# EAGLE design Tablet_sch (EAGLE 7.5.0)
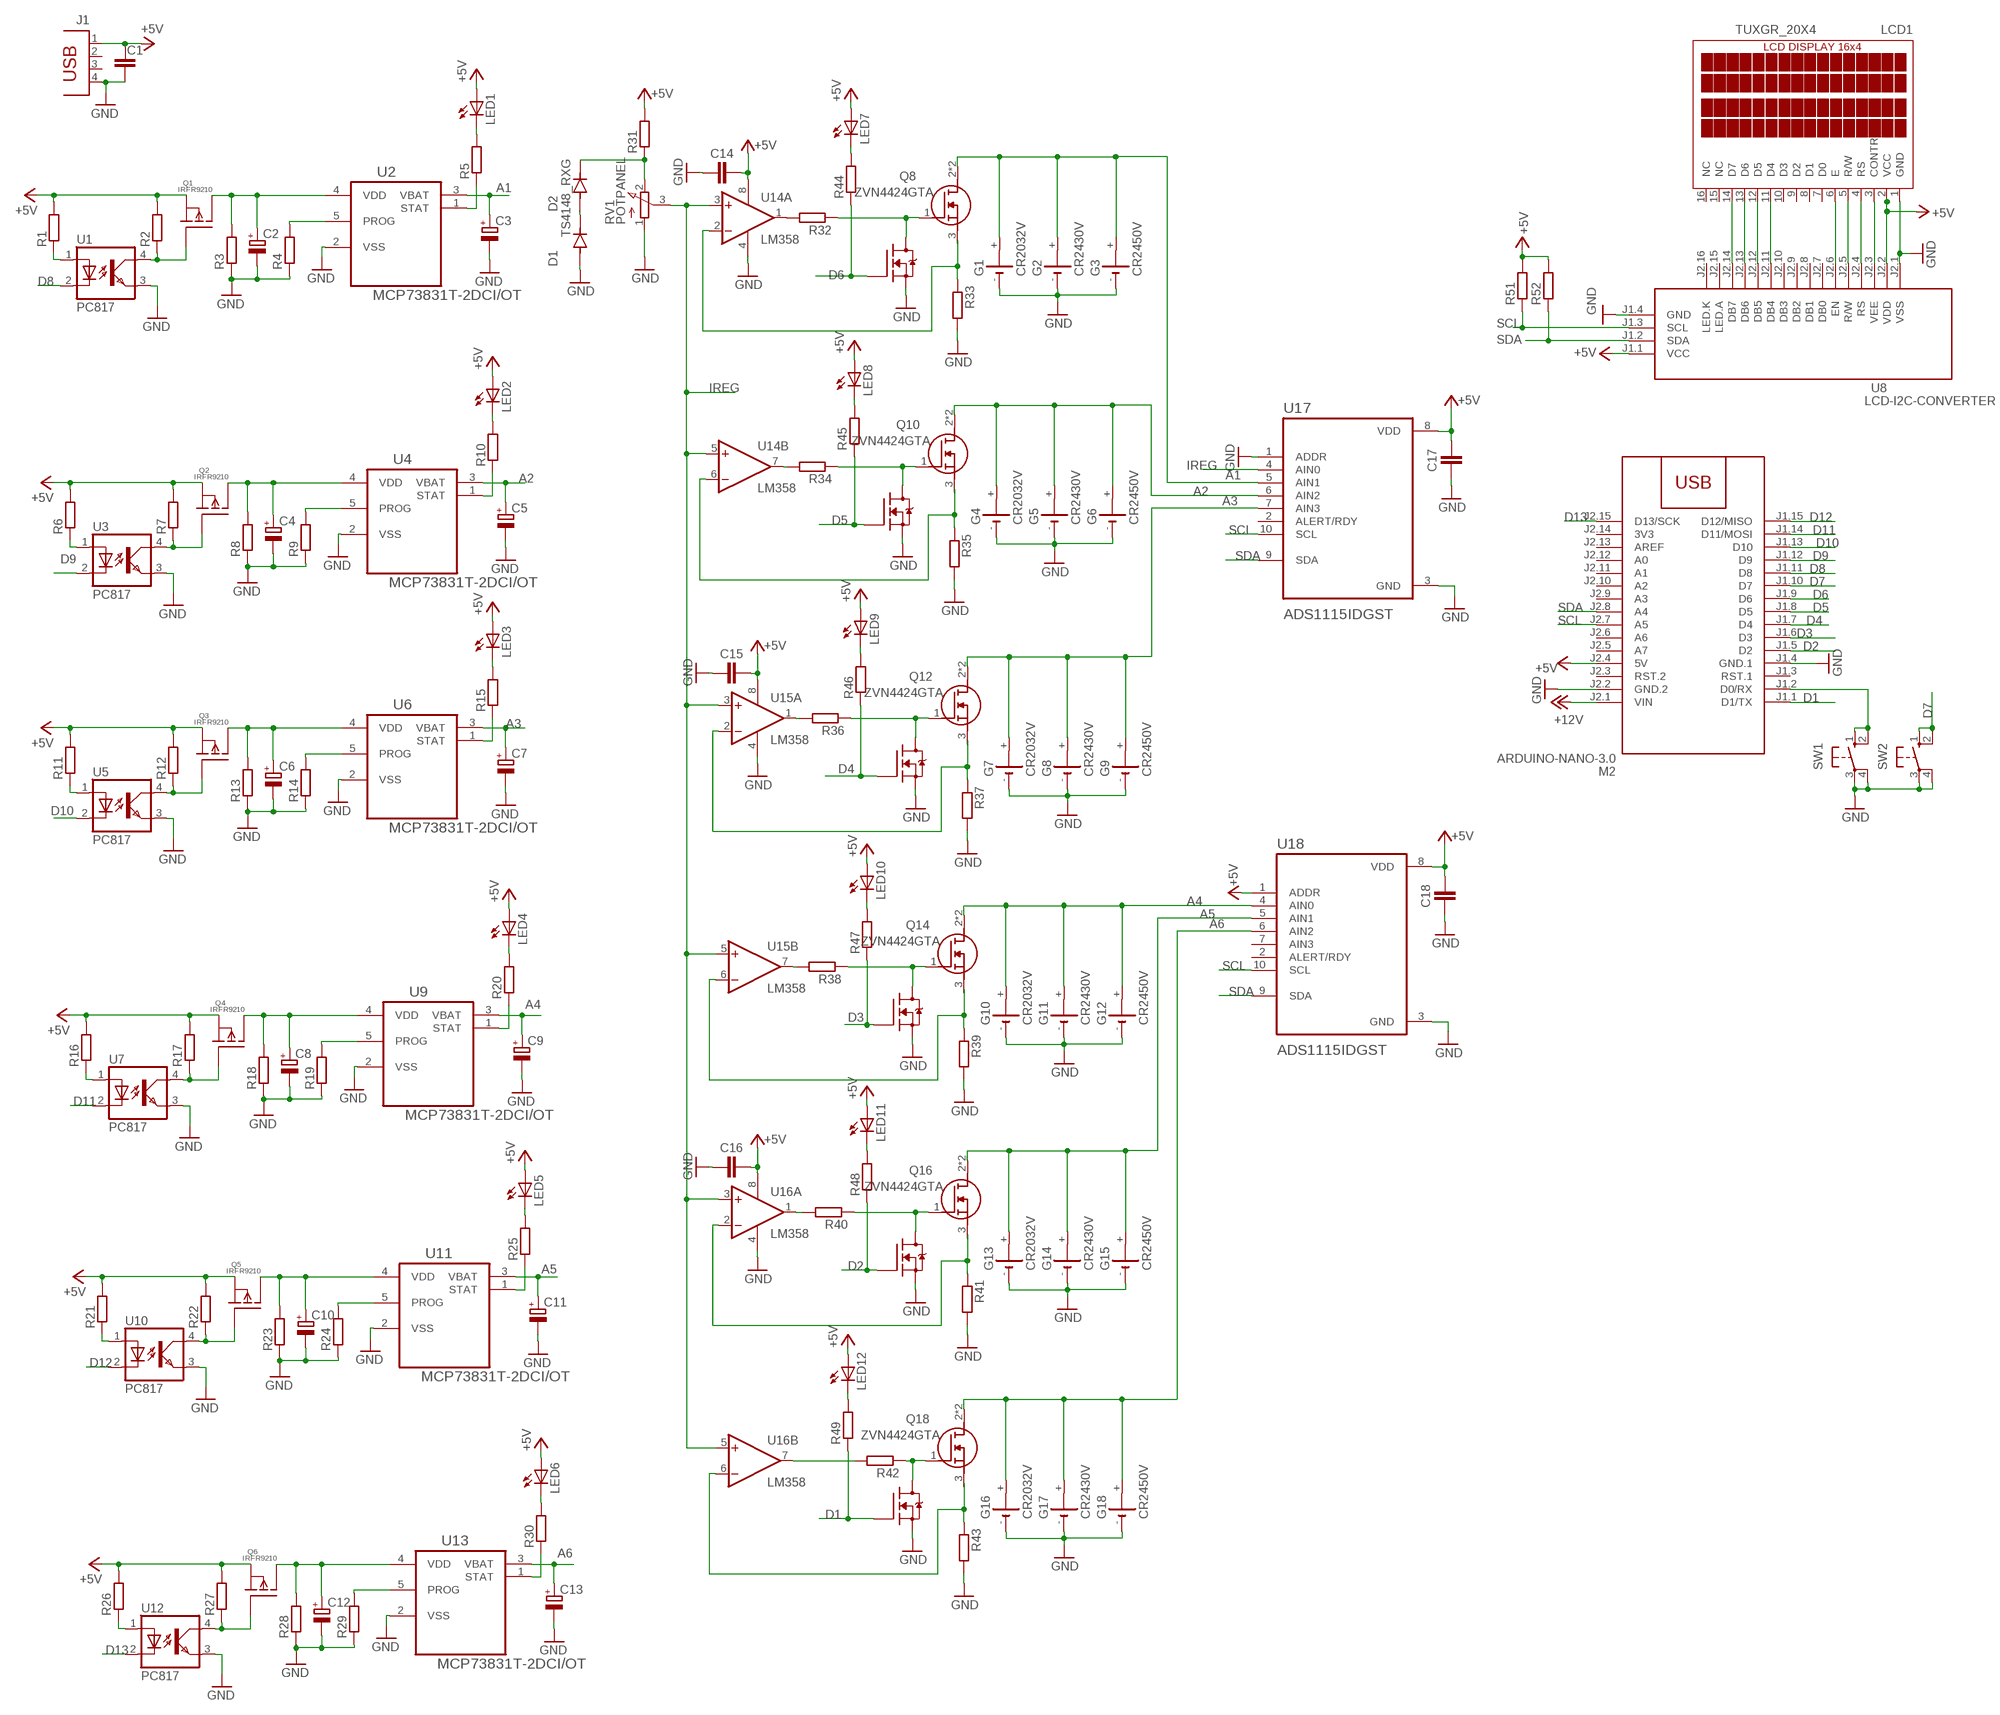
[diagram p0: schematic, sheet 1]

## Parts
C1  C-EUC1206  [C1206]
C2  CPOL-EUSMCB  [SMC_B]
C3  CPOL-EUSMCB  [SMC_B]
C4  CPOL-EUSMCB  [SMC_B]
C5  CPOL-EUSMCB  [SMC_B]
C6  CPOL-EUSMCB  [SMC_B]
C7  CPOL-EUSMCB  [SMC_B]
C8  CPOL-EUSMCB  [SMC_B]
C9  CPOL-EUSMCB  [SMC_B]
C10  CPOL-EUSMCB  [SMC_B]
C11  CPOL-EUSMCB  [SMC_B]
C12  CPOL-EUSMCB  [SMC_B]
C13  CPOL-EUSMCB  [SMC_B]
C14  C-EUC1206  [C1206]
C15  C-EUC1206  [C1206]
C16  C-EUC1206  [C1206]
C17  C-EUC1206  [C1206]
C18  C-EUC1206  [C1206]
D1  TS4148_RXG  [DIO_TS4148_RXG]
D2  TS4148_RXG  [DIO_TS4148_RXG]
G1  CR2032V  [CR2032V]
G2  CR2430V  [CR2430V]
G3  CR2450V  [CR2450V]
G4  CR2032V  [CR2032V]
G5  CR2430V  [CR2430V]
G6  CR2450V  [CR2450V]
G7  CR2032V  [CR2032V]
G8  CR2430V  [CR2430V]
G9  CR2450V  [CR2450V]
G10  CR2032V  [CR2032V]
G11  CR2430V  [CR2430V]
G12  CR2450V  [CR2450V]
G13  CR2032V  [CR2032V]
G14  CR2430V  [CR2430V]
G15  CR2450V  [CR2450V]
G16  CR2032V  [CR2032V]
G17  CR2430V  [CR2430V]
G18  CR2450V  [CR2450V]
J1  PN87520  [PN87520]
LCD1  TUXGR_20X4  [TUXGR_20X4]
LED1  LED5MM  [LED5MM]
LED2  LED5MM  [LED5MM]
LED3  LED5MM  [LED5MM]
LED4  LED5MM  [LED5MM]
LED5  LED5MM  [LED5MM]
LED6  LED5MM  [LED5MM]
LED7  LED5MM  [LED5MM]
LED8  LED5MM  [LED5MM]
LED9  LED5MM  [LED5MM]
LED10  LED5MM  [LED5MM]
LED11  LED5MM  [LED5MM]
LED12  LED5MM  [LED5MM]
M2  ARDUINO-NANO-3.0  [ARDUINO-NANO-3.0]
Q1  IRFR9210  [D2PACK]
Q2  IRFR9210  [D2PACK]
Q3  IRFR9210  [D2PACK]
Q4  IRFR9210  [D2PACK]
Q5  IRFR9210  [D2PACK]
Q6  IRFR9210  [D2PACK]
Q7  ZVN3310F  [SOT23]
Q8  ZVN4424GTA  [ZVN4424GTA]
Q9  ZVN3310F  [SOT23]
Q10  ZVN4424GTA  [ZVN4424GTA]
Q11  ZVN3310F  [SOT23]
Q12  ZVN4424GTA  [ZVN4424GTA]
Q13  ZVN3310F  [SOT23]
Q14  ZVN4424GTA  [ZVN4424GTA]
Q15  ZVN3310F  [SOT23]
Q16  ZVN4424GTA  [ZVN4424GTA]
Q17  ZVN3310F  [SOT23]
Q18  ZVN4424GTA  [ZVN4424GTA]
R1  R-EU_R1206  [R1206]
R2  R-EU_R1206  [R1206]
R3  R-EU_R1206  [R1206]
R4  R-EU_R1206  [R1206]
R5  R-EU_R1206  [R1206]
R6  R-EU_R1206  [R1206]
R7  R-EU_R1206  [R1206]
R8  R-EU_R1206  [R1206]
R9  R-EU_R1206  [R1206]
R10  R-EU_R1206  [R1206]
R11  R-EU_R1206  [R1206]
R12  R-EU_R1206  [R1206]
R13  R-EU_R1206  [R1206]
R14  R-EU_R1206  [R1206]
R15  R-EU_R1206  [R1206]
R16  R-EU_R1206  [R1206]
R17  R-EU_R1206  [R1206]
R18  R-EU_R1206  [R1206]
R19  R-EU_R1206  [R1206]
R20  R-EU_R1206  [R1206]
R21  R-EU_R1206  [R1206]
R22  R-EU_R1206  [R1206]
R23  R-EU_R1206  [R1206]
R24  R-EU_R1206  [R1206]
R25  R-EU_R1206  [R1206]
R26  R-EU_R1206  [R1206]
R27  R-EU_R1206  [R1206]
R28  R-EU_R1206  [R1206]
R29  R-EU_R1206  [R1206]
R30  R-EU_R1206  [R1206]
R31  R-EU_R1206  [R1206]
R32  R-EU_R1206  [R1206]
R33  R-EU_R2512  [R2512]
R34  R-EU_R1206  [R1206]
R35  R-EU_R2512  [R2512]
R36  R-EU_R1206  [R1206]
R37  R-EU_R2512  [R2512]
R38  R-EU_R1206  [R1206]
R39  R-EU_R2512  [R2512]
R40  R-EU_R1206  [R1206]
R41  R-EU_R2512  [R2512]
R42  R-EU_R1206  [R1206]
R43  R-EU_R2512  [R2512]
R44  R-EU_R1206  [R1206]
R45  R-EU_R1206  [R1206]
R46  R-EU_R1206  [R1206]
R47  R-EU_R1206  [R1206]
R48  R-EU_R1206  [R1206]
R49  R-EU_R1206  [R1206]
R51  R-EU_R1206  [R1206]
R52  R-EU_R1206  [R1206]
RV1  POTPANEL  [POTPANELP231]
SW1  40-XX  [B3F-40XX]
SW2  40-XX  [B3F-40XX]
U1  PC817  [DIL04]
U2  MCP73831T-2DCI/OT  [SOT95P270X145-5N]
U3  PC817  [DIL04]
U4  MCP73831T-2DCI/OT  [SOT95P270X145-5N]
U5  PC817  [DIL04]
U6  MCP73831T-2DCI/OT  [SOT95P270X145-5N]
U7  PC817  [DIL04]
U8  LCD-I2C-CONVERTER  [LCD-I2C-CONVERTER]
U9  MCP73831T-2DCI/OT  [SOT95P270X145-5N]
U10  PC817  [DIL04]
U11  MCP73831T-2DCI/OT  [SOT95P270X145-5N]
U12  PC817  [DIL04]
U13  MCP73831T-2DCI/OT  [SOT95P270X145-5N]
U14  LM358  OPA2134PA  [DIL08]
U15  LM358  OPA2134PA  [DIL08]
U16  LM358  OPA2134PA  [DIL08]
U17  ADS1115IDGST  [SOP50P490X110-10N]
U18  ADS1115IDGST  [SOP50P490X110-10N]

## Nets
+5V: C1.1 C14.1 C15.1 C16.1 C17.1 C18.1 J1.1 LCD1.2(VCC) LED1.A LED2.A LED3.A LED4.A LED5.A LED6.A LED7.A LED8.A LED9.A LED10.A LED11.A LED12.A M2.J2.4(5V) Q1.3(S) Q2.3(S) Q3.3(S) Q4.3(S) Q5.3(S) Q6.3(S) R1.2 R2.2 R6.2 R7.2 R11.2 R12.2 R16.2 R17.2 R21.2 R22.2 R26.2 R27.2 R31.2 R51.2 R52.2 U8.J1.1(VCC) U8.J2.2(VDD) U14.8(A:V+) U15.8(A:V+) U16.8(A:V+) U17.8(VDD) U18.1(ADDR) U18.8(VDD)
+12V: M2.J2.1(VIN)
A1: C3.+ G1.+ G2.+ G3.+ Q8.2(D) Q8.4(D) U2.3(VBAT) U17.5(AIN1)
A2: C5.+ G4.+ G5.+ G6.+ Q10.2(D) Q10.4(D) U4.3(VBAT) U17.6(AIN2)
A3: C7.+ G7.+ G8.+ G9.+ Q12.2(D) Q12.4(D) U6.3(VBAT) U17.7(AIN3)
A4: C9.+ G10.+ G11.+ G12.+ Q14.2(D) Q14.4(D) U9.3(VBAT) U18.4(AIN0)
A5: C11.+ G13.+ G14.+ G15.+ Q16.2(D) Q16.4(D) U11.3(VBAT) U18.5(AIN1)
A6: C13.+ G16.+ G17.+ G18.+ Q18.2(D) Q18.4(D) U13.3(VBAT) U18.6(AIN2)
D1: M2.J1.1(D1/TX) Q17.2(G) R49.1
D2: M2.J1.5(D2) Q15.2(G) R48.1
D3: M2.J1.6(D3) Q13.2(G) R47.1
D4: M2.J1.7(D4) Q11.2(G) R46.1
D5: M2.J1.8(D5) Q9.2(G) R45.1
D6: M2.J1.9(D6) Q7.2(G) R44.1
D7: M2.J1.10(D7) SW2.1(S) SW2.2(S1)
D8: M2.J1.11(D8) U1.2(C)
D9: M2.J1.12(D9) U3.2(C)
D10: M2.J1.13(D10) U5.2(C)
D11: M2.J1.14(D11/MOSI) U7.2(C)
D12: M2.J1.15(D12/MISO) U10.2(C)
D13: M2.J2.15(D13/SCK) U12.2(C)
GND: C1.2 C2.- C3.- C4.- C5.- C6.- C7.- C8.- C9.- C10.- C11.- C12.- C13.- C14.2 C15.2 C16.2 C17.2 C18.2 D1.A G1.- G2.- G3.- G4.- G5.- G6.- G7.- G8.- G9.- G10.- G11.- G12.- G13.- G14.- G15.- G16.- G17.- G18.- J1.4 LCD1.1(GND) M2.J1.4(GND.1) M2.J2.2(GND.2) Q7.3(S) Q9.3(S) Q11.3(S) Q13.3(S) Q15.3(S) Q17.3(S) R3.1 R4.1 R8.1 R9.1 R13.1 R14.1 R18.1 R19.1 R23.1 R24.1 R28.1 R29.1 R33.2 R35.2 R37.2 R39.2 R41.2 R43.2 RV1.1(A) SW1.3(P) SW1.4(P1) SW2.3(P) SW2.4(P1) U1.3(EMIT) U2.2(VSS) U3.3(EMIT) U4.2(VSS) U5.3(EMIT) U6.2(VSS) U7.3(EMIT) U8.J1.4(GND) U8.J2.1(VSS) U9.2(VSS) U10.3(EMIT) U11.2(VSS) U12.3(EMIT) U13.2(VSS) U14.4(A:V-) U15.4(A:V-) U16.4(A:V-) U17.1(ADDR) U17.3(GND) U18.3(GND)
IREG: RV1.3(S) U14.3(A:+IN) U14.5(B:+IN) U15.3(A:+IN) U15.5(B:+IN) U16.3(A:+IN) U16.5(B:+IN) U17.4(AIN0)
N$1: LCD1.14(D7) U8.J2.14(DB7)
N$2: LCD1.13(D6) U8.J2.13(DB6)
N$3: LCD1.12(D5) U8.J2.12(DB5)
N$4: LCD1.11(D4) U8.J2.11(DB4)
N$5: LCD1.6(E) U8.J2.6(EN)
N$6: LCD1.5(R/W) U8.J2.5(R/W)
N$7: LCD1.4(RS) U8.J2.4(RS)
N$8: M2.J1.2(D0/RX) SW1.1(S) SW1.2(S1)
N$9: R1.1 U1.1(A)
N$10: LCD1.3(CONTR) U8.J2.3(VEE)
N$11: LED6.K(C) R30.2
N$12: Q1.1(G) R2.1 U1.4(COL)
N$13: C2.+ Q1.2(D) R3.2 U2.4(VDD)
N$14: R5.1 U2.1(STAT)
N$15: R4.2 U2.5(PROG)
N$16: LED1.K(C) R5.2
N$18: R6.1 U3.1(A)
N$20: Q2.1(G) R7.1 U3.4(COL)
N$21: C4.+ Q2.2(D) R8.2 U4.4(VDD)
N$22: R9.2 U4.5(PROG)
N$24: R10.1 U4.1(STAT)
N$25: LED2.K(C) R10.2
N$26: R11.1 U5.1(A)
N$28: Q3.1(G) R12.1 U5.4(COL)
N$29: C6.+ Q3.2(D) R13.2 U6.4(VDD)
N$30: R14.2 U6.5(PROG)
N$32: R15.1 U6.1(STAT)
N$33: LED3.K(C) R15.2
N$34: R16.1 U7.1(A)
N$36: Q4.1(G) R17.1 U7.4(COL)
N$37: C8.+ Q4.2(D) R18.2 U9.4(VDD)
N$38: R19.2 U9.5(PROG)
N$40: R20.1 U9.1(STAT)
N$41: LED4.K(C) R20.2
N$42: R21.1 U10.1(A)
N$44: Q5.1(G) R22.1 U10.4(COL)
N$45: C10.+ Q5.2(D) R23.2 U11.4(VDD)
N$46: R24.2 U11.5(PROG)
N$48: R25.1 U11.1(STAT)
N$49: LED5.K(C) R25.2
N$50: R26.1 U12.1(A)
N$52: Q6.1(G) R27.1 U12.4(COL)
N$53: C12.+ Q6.2(D) R28.2 U13.4(VDD)
N$54: R29.2 U13.5(PROG)
N$56: R30.1 U13.1(STAT)
N$58: D2.C(K) R31.1 RV1.2(E)
N$59: D1.C(K) D2.A
N$60: R32.2 U14.1(A:OUT)
N$61: Q7.1(D) Q8.1(G) R32.1
N$62: Q8.3(S) R33.1 U14.2(A:-IN)
N$64: R34.2 U14.7(B:OUT)
N$65: Q9.1(D) Q10.1(G) R34.1
N$66: Q10.3(S) R35.1 U14.6(B:-IN)
N$68: R36.2 U15.1(A:OUT)
N$69: Q11.1(D) Q12.1(G) R36.1
N$70: Q12.3(S) R37.1 U15.2(A:-IN)
N$72: R38.2 U15.7(B:OUT)
N$73: Q13.1(D) Q14.1(G) R38.1
N$74: Q14.3(S) R39.1 U15.6(B:-IN)
N$76: R40.2 U16.1(A:OUT)
N$77: Q15.1(D) Q16.1(G) R40.1
N$78: Q16.3(S) R41.1 U16.2(A:-IN)
N$80: R42.2 U16.7(B:OUT)
N$81: Q17.1(D) Q18.1(G) R42.1
N$82: Q18.3(S) R43.1 U16.6(B:-IN)
N$84: LED8.K(C) R45.2
N$85: LED10.K(C) R47.2
N$86: LED11.K(C) R48.2
N$87: LED12.K(C) R49.2
N$90: LED9.K(C) R46.2
N$91: LED7.K(C) R44.2
SCL: M2.J2.7(A5) R51.1 U8.J1.3(SCL) U17.10(SCL) U18.10(SCL)
SDA: M2.J2.8(A4) R52.1 U8.J1.2(SDA) U17.9(SDA) U18.9(SDA)
Unconnected: G1.+@1(+) G2.+@1(+) G3.+@1(+) G4.+@1(+) G5.+@1(+) G6.+@1(+) G7.+@1(+) G8.+@1(+) G9.+@1(+) G10.+@1(+) G11.+@1(+) G12.+@1(+) G13.+@1(+) G14.+@1(+) G15.+@1(+) G16.+@1(+) G17.+@1(+) G18.+@1(+) J1.2 J1.3 LCD1.7(D0) LCD1.8(D1) LCD1.9(D2) LCD1.10(D3) LCD1.15(NC) LCD1.16(NC) M2.J1.3(RST.1) M2.J2.3(RST.2) M2.J2.5(A7) M2.J2.6(A6) M2.J2.9(A3) M2.J2.10(A2) M2.J2.11(A1) M2.J2.12(A0) M2.J2.13(AREF) U8.J2.7(DB0) U8.J2.8(DB1) U8.J2.9(DB2) U8.J2.10(DB3) U8.J2.15(LED.A) U8.J2.16(LED.K) U17.2(ALERT/RDY) U18.2(ALERT/RDY) U18.7(AIN3)

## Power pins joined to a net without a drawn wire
3V3: M2.J2.14(3V3)

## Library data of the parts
C1 C14-C18 = rcl:C-EU: CAPACITOR, European symbol
C2-C13 = rcl:CPOL-EU: POLARIZED CAPACITOR, European symbol
D1 D2 = TS4148_RXG:TS4148_RXG: Check availability Check availability Check availability; AVAILABILITY: In Stock; CHECK_PRICES: https://www.snapeda.com/parts/TS4148%20RXG/Taiwan+Semiconductor/view-part/?ref=eda; DESCRIPTION: 1206 (Ceramics) 75V 0.15A Switching Diode & Array; MF: Taiwan Semiconductor; MP: TS4148 RXG; PACKAGE: 1206-2 Taiwan Semiconductor; PRICE: None; SNAPEDA_LINK: https://www.snapeda.com/parts/TS4148%20RXG/Taiwan+Semiconductor/view-part/?ref=snap
G1 G4 G7 G10 G13 G16 = battery:CR2032V: LI BATTERY Varta
G2 G5 G8 G11 G14 G17 = battery:CR2430V: LI BATTERY Varta
G3 G6 G9 G12 G15 G18 = battery:CR2450V: LI BATTERY Varta
J1 = con-berg:PN87520: BERG USB connector; OC_FARNELL: unknown; OC_NEWARK: unknown
LCD1 = display-lcd:TUXGR_20X4: LCD DISPLAY 20X4
LED1-LED12 = led:LED: LED
M2 = diy-modules:ARDUINO-NANO-3.0: Arduino Nano 3.0 and compatible devices More details available here: https://www.arduino.cc/en/Main/ArduinoBoardNano Click here to find device on ebay.com
Q1-Q6 = IRFR9210:IRFR9210: Check availability; AVAILABILITY: In Stock; CHECK_PRICES: https://www.snapeda.com/parts/IRFR9210/Vishay+Siliconix/view-part/?ref=eda; DESCRIPTION: P-Channel 200 V 1.9A (Tc) 2.5W (Ta), 25W (Tc) Surface Mount D-Pak; MF: Vishay; MP: IRFR9210; PACKAGE: TO-252-3 Infineon; PRICE: None; SNAPEDA_LINK: https://www.snapeda.com/parts/IRFR9210/Vishay+Siliconix/view-part/?ref=snap
Q7 Q9 Q11 Q13 Q15 Q17 = transistor-fet:ZVN3310F
Q8 Q10 Q12 Q14 Q16 Q18 = ZVN4424GTA:ZVN4424GTA: Check availability; AVAILABILITY: In Stock; CHECK_PRICES: https://www.snapeda.com/parts/ZVN4424GTA/Diodes+Inc./view-part/?ref=eda; DESCRIPTION: Trans MOSFET N-CH 240V 0.5A 4-Pin(3+Tab) SOT-223 T/R; MF: Diodes Zetex; MP: ZVN4424GTA; PACKAGE: None; PRICE: None; SNAPEDA_LINK: https://www.snapeda.com/parts/ZVN4424GTA/Diodes+Inc./view-part/?ref=snap
R1-R49 R51 R52 = rcl:R-EU_: RESISTOR, European symbol
RV1 = pot:POTPANEL
SW1 SW2 = switch-omron:40-XX: OMRON SWITCH; MF: OMRON COMPONENTS USA; MPN: B3F-4000; OC_FARNELL: 176434; OC_NEWARK: 36K3105
U1 U3 U5 U7 U10 U12 = optocoupler:PC817: SHARP OPTO COUPLER; MPN: PC817X4J000F; OC_FARNELL: 9707727; OC_NEWARK: 97K7059
U2 U4 U6 U9 U11 U13 = MCP73831T-2DCI_OT:MCP73831T-2DCI/OT: Check availability; AVAILABILITY: In Stock; CHECK_PRICES: https://www.snapeda.com/parts/MCP73831T-2DCI/OT/Microchip+Technology/view-part/?ref=eda; DESCRIPTION: Microchip MCP73831T-2DCI/OT, Battery Charge Controller, 500mA, 5-Pin SOT-23 | Microchip Technology Inc. MCP73831T-2DCI/OT; MF: Microchip; MP: MCP73831T-2DCI/OT; PACKAGE: SOT-23-5 Microchip; PRICE: None; SNAPEDA_LINK: https://www.snapeda.com/parts/MCP73831T-2DCI/OT/Microchip+Technology/view-part/?ref=snap
U8 = diy-modules:LCD-I2C-CONVERTER: I2C Bus to 4-Bit Parallel LCD Interface with LED backlight driver
U14-U16 = linear:OPA2*: Dual Operational Amplifier Low Power, Single-Supply, Rail-To-Rail Operational Amplifier Source: http://focus.ti.com/lit/ds/symlink/opa2345.pdf http://focus.ti.com .. opa241.pdf http://focus.ti.com/lit/ds/symlink/opa2134.pdf
U17 U18 = ADS1115IDGST:ADS1115IDGST: Check availability; AVAILABILITY: In Stock; CHECK_PRICES: https://www.snapeda.com/parts/ADS1115IDGST/Texas+Instruments/view-part/?ref=eda; DESCRIPTION: 16-bit, 860-SPS, 4-channel, delta-sigma ADC with PGA, oscillator, VREF, comparator and I2C; MF: Texas Instruments; MP: ADS1115IDGST; PACKAGE: VSSOP-10 Texas Instruments; PRICE: None; SNAPEDA_LINK: https://www.snapeda.com/parts/ADS1115IDGST/Texas+Instruments/view-part/?ref=snap

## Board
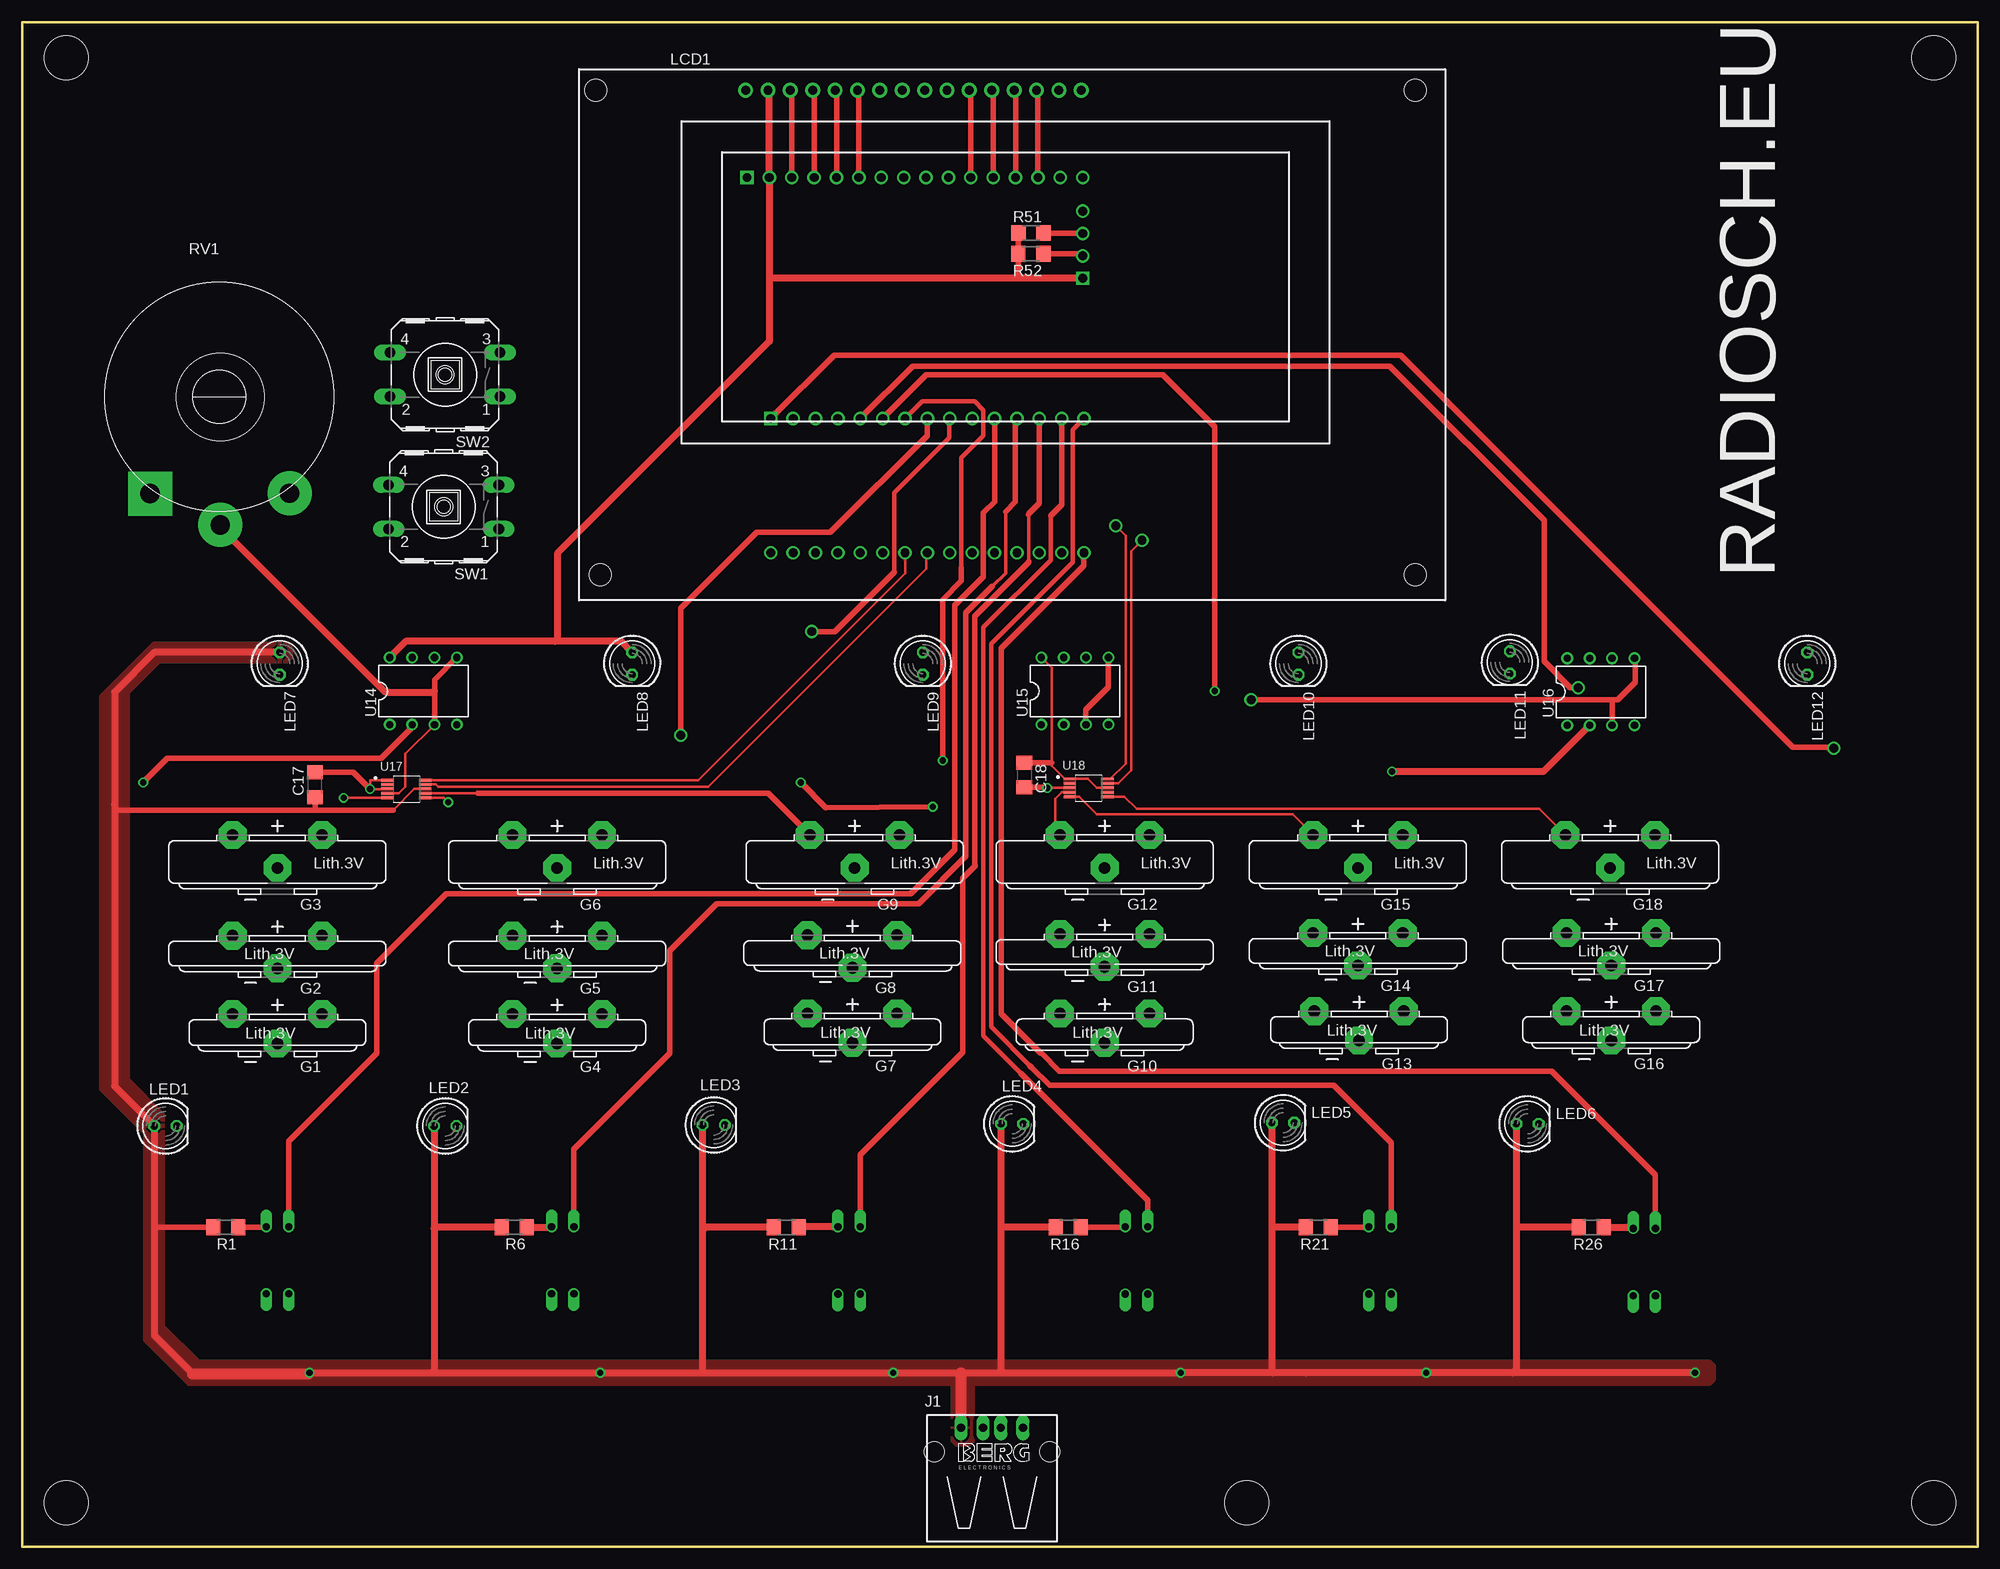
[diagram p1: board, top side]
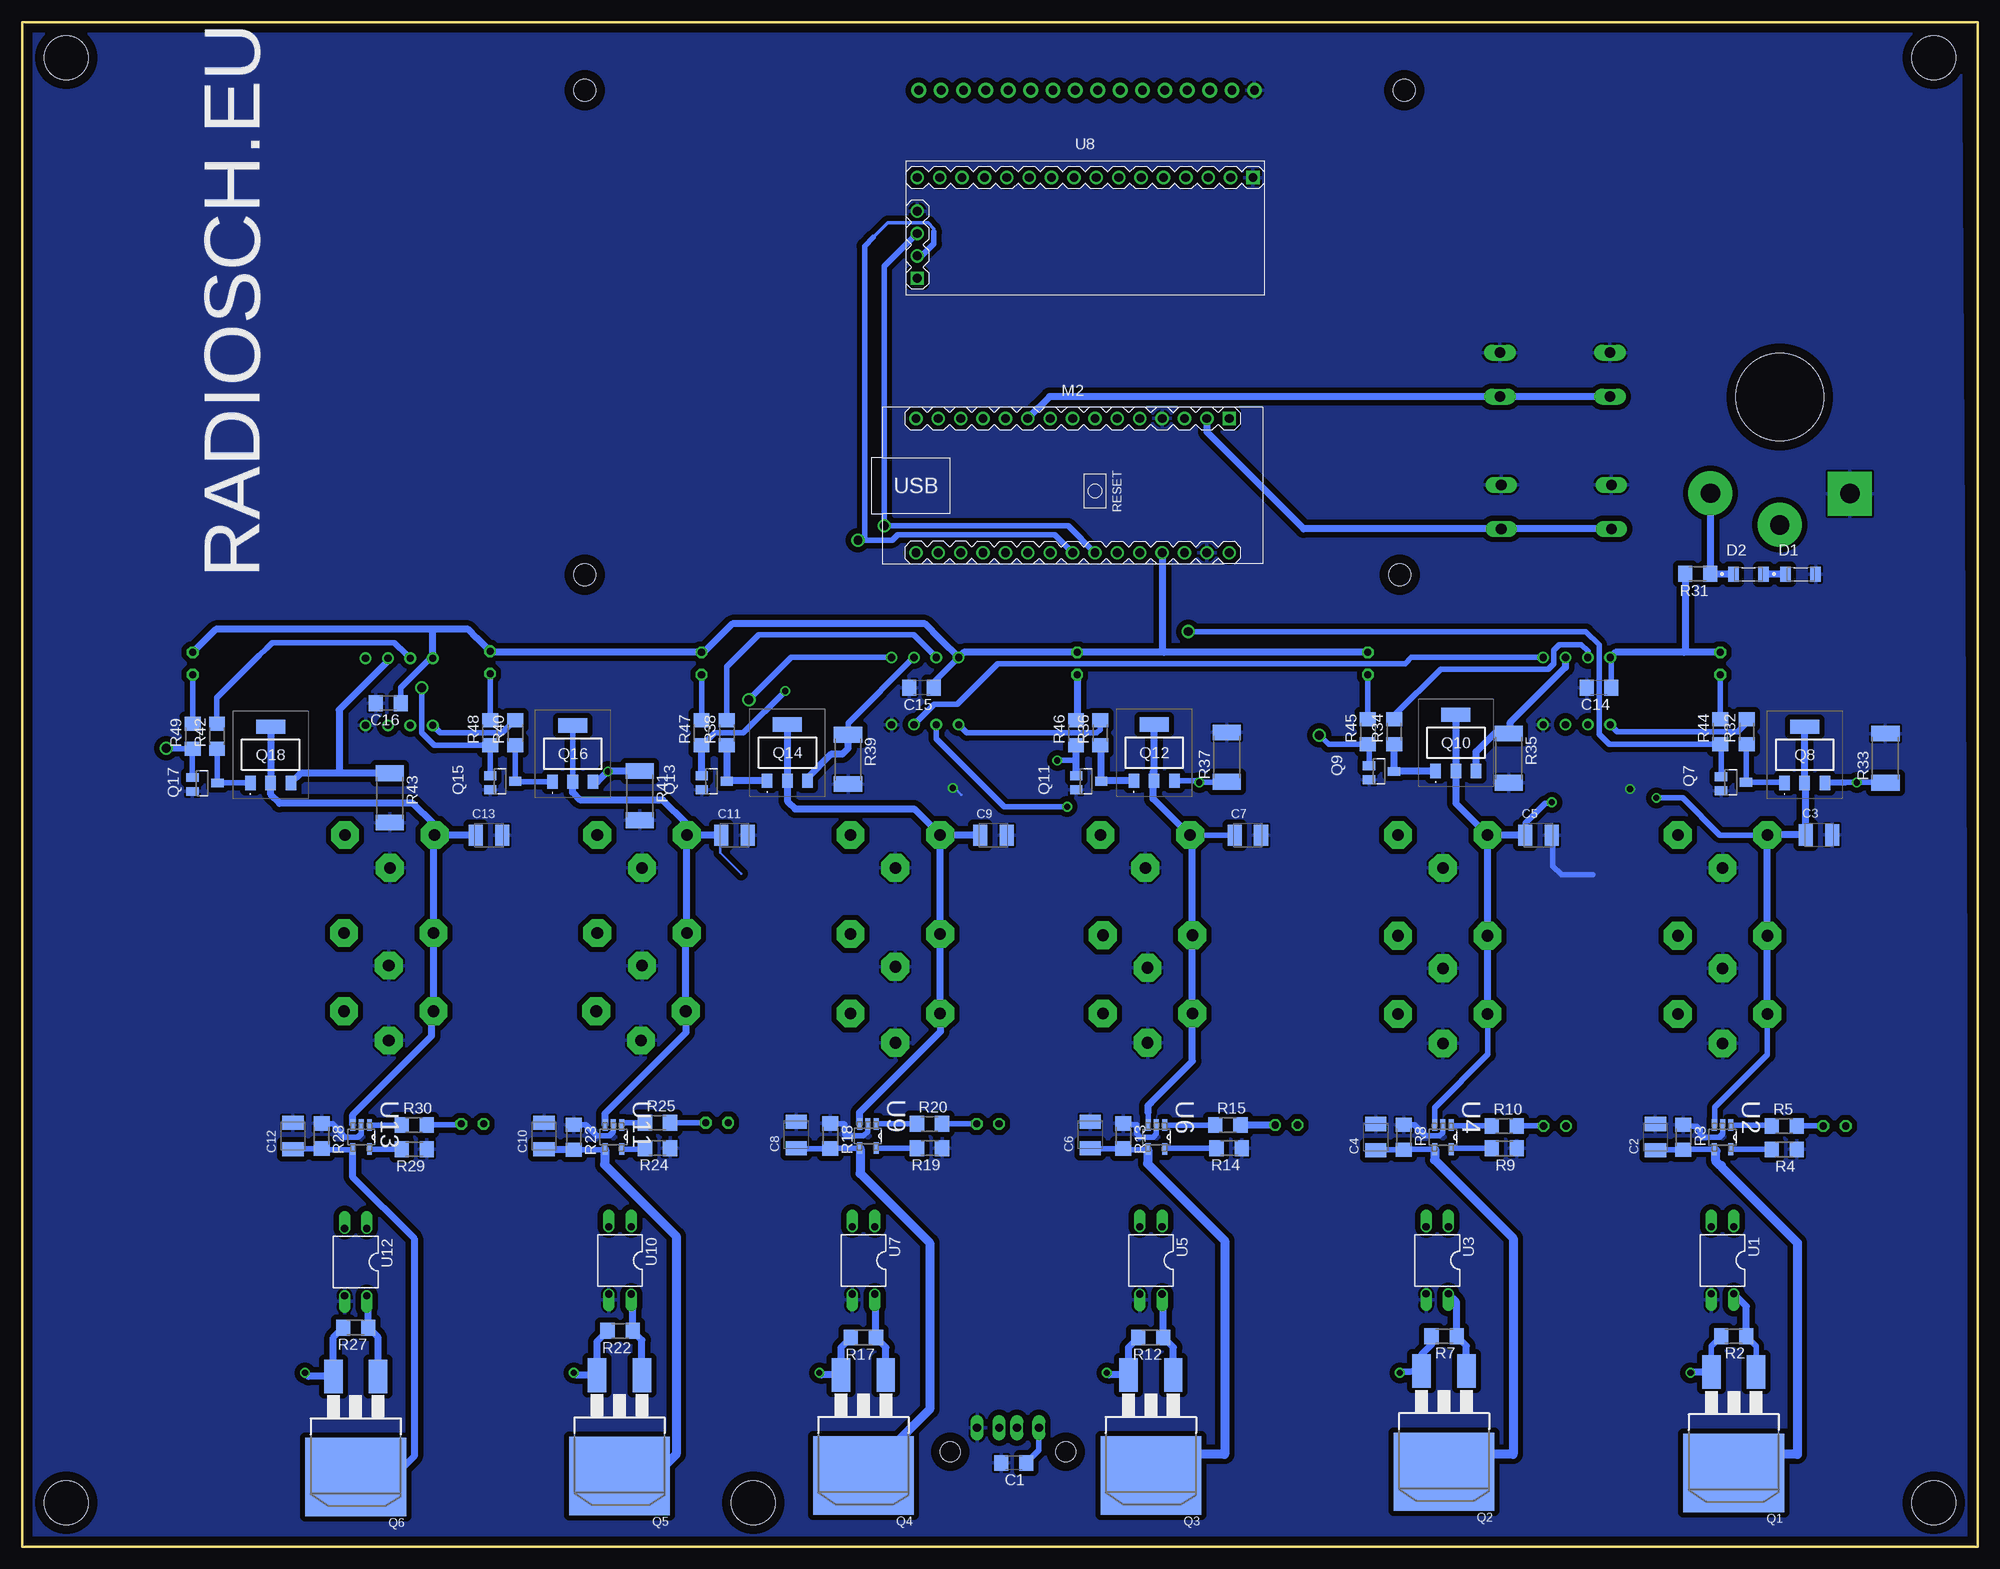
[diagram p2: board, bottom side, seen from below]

Size 222 x 173.06 mm. Coordinates in mm from the lower left corner, seen from the top.
Outline: 0,0 222,0 222,173.06 0,173.06 0,0
Copper layers (1*16): Top 0.035mm / dielectric 1.5mm / Bottom 0.035mm
Design rules "default": minimum track width 10mil, minimum drill 24mil, track to track 8mil, track to pad 8mil, pad to pad 8mil, via to via 8mil, smd to smd 8mil, copper to edge 40mil, drill to drill 8mil, minimum pad ring 10mil, minimum via ring 8mil, stop-mask expansion 4mil, vias tented up to drill 0mil, thermal gap 10mil
Holes 10 mm at 22.5,130.5
Holes 5 mm at 5,169 5,5 139,5 217,5 217,169

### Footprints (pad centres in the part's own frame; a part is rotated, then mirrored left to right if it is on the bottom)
C1206 = smd 1.6 x 1.8: 1 -1.4,0; 2 1.4,0
SMC_B = smd 1.6 x 2.4: + -1.5,0; - 1.5,0
DIO_TS4148_RXG = smd 1.2 x 1.7: A 1.7,0; C -1.7,0
CR2032V = drill 1.321 pad 3.15 octagon: + -2.54,-5.08; +@1 -2.54,5.08; - 0.786,0
CR2430V = drill 1.321 pad 3.15 octagon: + -2.54,-5.08; +@1 -2.54,5.08; - 1.159,0
CR2450V = drill 1.321 pad 3.15 octagon: + -2.54,-5.08; +@1 -2.54,5.08; - 1.191,0
PN87520 = drill 0.95 long: 1 -3.5,2.71; 2 -1,2.71; 3 1,2.71; 4 3.5,2.71 | hole 2.3: -6.57,0; 6.57,0
TUXGR_20X4 = drill 1 pad 1.676: 1 11.14,-2.28; 2 13.68,-2.28; 3 16.22,-2.28; 4 18.76,-2.28; 5 21.3,-2.28; 6 23.84,-2.28; 7 26.38,-2.28; 8 28.92,-2.28; 9 31.46,-2.28; 10 34,-2.28; 11 36.54,-2.28; 12 39.08,-2.28; 13 41.62,-2.28; 14 44.16,-2.28; 15 46.7,-2.28; 16 49.24,-2.28 | hole 2.5: -5.36,-57.28; 87.14,-57.28; -5.86,-2.28; 87.14,-2.28
LED5MM = drill 0.813 octagon: A -1.27,0; K 1.27,0
ARDUINO-NANO-3.0 = drill 1 square: J1.1 17.78,7.62 | drill 1: J1.2 15.24,7.62; J1.3 12.7,7.62; J1.4 10.16,7.62; J1.5 7.62,7.62; J1.6 5.08,7.62; J1.7 2.54,7.62; J1.8 0,7.62; J1.9 -2.54,7.62; J1.10 -5.08,7.62; J1.11 -7.62,7.62; J1.12 -10.16,7.62; J1.13 -12.7,7.62; J1.14 -15.24,7.62; J1.15 -17.78,7.62; J2.1 17.78,-7.62; J2.2 15.24,-7.62; J2.3 12.7,-7.62; J2.4 10.16,-7.62; J2.5 7.62,-7.62; J2.6 5.08,-7.62; J2.7 2.54,-7.62; J2.8 0,-7.62; J2.9 -2.54,-7.62; J2.10 -5.08,-7.62; J2.11 -7.62,-7.62; J2.12 -10.16,-7.62; J2.13 -12.7,-7.62; J2.14 -15.24,-7.62; J2.15 -17.78,-7.62
D2PACK = smd 2.083 x 3.81: 1 -2.54,-8.89; 3 2.54,-8.89 | smd 11.43 x 8.89: 2 0,2.54
SOT23 = smd 1 x 1.4: 1 0,1.735; 2 -0.632,-1.1; 3 0.95,-1.1
ZVN4424GTA = smd 1.2 x 1.6: 1 -2.3,-3.2; 2 0,-3.2; 3 2.3,-3.2 | smd 3.3 x 1.6: 4 0,3.2
R1206 = smd 1.6 x 1.803: 1 -1.422,0; 2 1.422,0
R2512 = smd 1.8 x 3.2: 1 -2.8,0; 2 2.8,0
POTPANELP231 = drill 2.2 pad 5 square: 1 -7.85,-11 | drill 2.2 pad 5: 2 7.97,-10.96; 3 0.11,-14.54
B3F-40XX = drill 1.194 long: 1 -6.248,2.489; 2 6.248,2.489; 3 -6.248,-2.489; 4 6.248,-2.489
DIL04 = drill 0.813 offset: 1 -1.27,-3.81; 2 1.27,-3.81; 3 1.27,3.81; 4 -1.27,3.81
SOT95P270X145-5N = smd 1.321 x 0.559: 1 -1.372,0.94; 2 -1.372,0; 3 -1.372,-0.94; 4 1.372,-0.94; 5 1.372,0.94
LCD-I2C-CONVERTER = drill 1 square: J1.1 -19.05,-5.08; J2.1 19.05,6.35 | drill 1: J1.2 -19.05,-2.54; J1.3 -19.05,0; J1.4 -19.05,2.54; J2.2 16.51,6.35; J2.3 13.97,6.35; J2.4 11.43,6.35; J2.5 8.89,6.35; J2.6 6.35,6.35; J2.7 3.81,6.35; J2.8 1.27,6.35; J2.9 -1.27,6.35; J2.10 -3.81,6.35; J2.11 -6.35,6.35; J2.12 -8.89,6.35; J2.13 -11.43,6.35; J2.14 -13.97,6.35; J2.15 -16.51,6.35; J2.16 -19.05,6.35
DIL08 = drill 0.813 pad 1.27: 1 -3.81,-3.81; 2 -1.27,-3.81; 3 1.27,-3.81; 4 3.81,-3.81; 5 3.81,3.81; 6 1.27,3.81; 7 -1.27,3.81; 8 -3.81,3.81
SOP50P490X110-10N = smd 1.47 x 0.28: 1 -2.15,1; 2 -2.15,0.5; 3 -2.15,0; 4 -2.15,-0.5; 5 -2.15,-1; 6 2.15,-1; 7 2.15,-0.5; 8 2.15,0; 9 2.15,0.5; 10 2.15,1

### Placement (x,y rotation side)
C1  109.44,9.51 180 bottom
C2  36.6,46.49 90 bottom
C3  18.02,80.8 0 bottom
C4  68.36,46.49 90 bottom
C5  49.88,80.75 0 bottom
C6  100.75,46.75 90 bottom
C7  82.88,80.75 0 bottom
C8  134.12,46.75 90 bottom
C9  111.75,80.75 0 bottom
C10  162.75,46.62 90 bottom
C11  141.12,80.75 0 bottom
C12  191.25,46.62 90 bottom
C13  169,80.75 0 bottom
C14  43.02,97.51 180 bottom
C15  119.9,97.49 180 bottom
C16  180.43,95.76 180 bottom
C17  33.26,86.49 90 top
C18  113.74,87.59 270 top
D1  20.12,110.39 0 bottom
D2  26.05,110.39 0 bottom
G1  28.98,57.92 270 top
G2  28.98,66.81 270 top
G3  28.98,78.24 270 top
G4  60.73,57.92 270 top
G5  60.73,66.81 270 top
G6  60.73,78.24 270 top
G7  94.25,58 270 top
G8  94.25,66.88 270 top
G9  94.5,78.25 270 top
G10  122.88,58 270 top
G11  122.88,67 270 top
G12  122.88,78.25 270 top
G13  151.75,58.25 270 top
G14  151.62,67.12 270 top
G15  151.62,78.25 270 top
G16  180.38,58.25 270 top
G17  180.38,67.12 270 top
G18  180.25,78.25 270 top
J1  110.09,10.8 0 top
LCD1  70.98,167.59 0 top
LED1  16.29,47.76 0 top
LED2  48.03,47.76 0 top
LED3  78.5,47.88 0 top
LED4  112.38,48 0 top
LED5  143.12,48.12 0 top
LED6  170.88,48 0 top
LED7  29.25,100.25 270 top
LED8  69.25,100.25 270 top
LED9  102.25,100.25 270 top
LED10  144.88,100.25 270 top
LED11  168.88,100.38 270 top
LED12  202.62,100.25 270 top
M2  102.76,120.45 0 bottom
Q1  27.71,10.93 180 bottom
Q2  60.61,11.05 180 bottom
Q3  93.88,10.62 180 bottom
Q4  126.5,10.62 180 bottom
Q5  154.19,10.58 180 bottom
Q6  184.12,10.46 180 bottom
Q7  28.06,86.77 270 bottom
Q8  19.66,89.89 0 bottom
Q9  68,88 270 bottom
Q10  59.25,91.25 0 bottom
Q11  101.25,86.88 270 bottom
Q12  93.5,90.12 0 bottom
Q13  143.75,86.88 270 bottom
Q14  135.12,90.12 0 bottom
Q15  167.75,86.88 270 bottom
Q16  159.49,90.02 0 bottom
Q17  201.56,86.68 270 bottom
Q18  193.79,89.89 0 bottom
R1  23.11,36.27 180 top
R2  27.71,23.9 180 bottom
R3  33.43,46.49 270 bottom
R4  22,45.09 180 bottom
R5  22,47.76 0 bottom
R6  55.87,36.27 180 top
R7  60.6,23.9 180 bottom
R8  65.18,46.49 270 bottom
R9  53.75,45.22 180 bottom
R10  53.75,47.76 0 bottom
R11  86.75,36.25 180 top
R12  93.88,23.75 180 bottom
R13  97,46.62 270 bottom
R14  85,45.25 180 bottom
R15  85.12,47.88 0 bottom
R16  118.75,36.25 180 top
R17  126.5,23.75 180 bottom
R18  130.25,46.62 270 bottom
R19  119,45.25 180 bottom
R20  119,48 0 bottom
R21  147.12,36.25 180 top
R22  154.12,24.5 180 bottom
R23  159.38,46.5 270 bottom
R24  149.88,45.25 180 bottom
R25  149.88,48.12 0 bottom
R26  178.12,36.25 180 top
R27  184.12,24.88 180 bottom
R28  188,46.62 270 bottom
R29  177.5,45.12 180 bottom
R30  177.5,47.88 0 bottom
R31  31.82,110.43 180 bottom
R32  26.25,92.5 90 bottom
R33  10.5,89.5 90 bottom
R34  66.25,92.5 90 bottom
R35  53.25,89.5 270 bottom
R36  99.62,92.38 90 bottom
R37  85.25,89.62 90 bottom
R38  142,92.38 90 bottom
R39  128.25,89.38 270 bottom
R40  166,92.38 90 bottom
R41  151.88,85.25 270 bottom
R42  199.88,92 90 bottom
R43  180.25,85 270 bottom
R44  29.25,92.5 90 bottom
R45  69.25,92.5 90 bottom
R46  102.38,92.38 90 bottom
R47  144.88,92.38 90 bottom
R48  168.88,92.38 90 bottom
R49  202.62,92 90 bottom
R51  114.52,149.11 180 top
R52  114.51,146.76 180 top
RV1  22.39,130.53 0 top
SW1  47.86,118.03 180 top
SW2  48.02,133.03 180 top
U1  28.98,32.52 180 bottom
U2  28.98,46.49 270 bottom
U3  61.37,32.52 180 bottom
U4  60.73,46.49 270 bottom
U5  93.88,32.5 180 bottom
U6  93.25,46.5 270 bottom
U7  126.5,32.5 180 bottom
U8  101.33,149.06 0 bottom
U9  126,46.62 270 bottom
U10  154.12,32.5 180 bottom
U11  154.88,46.5 270 bottom
U12  184.12,32.32 180 bottom
U13  183.5,46.5 270 bottom
U14  45.55,97.13 0 top
U15  119.5,97.12 0 top
U16  179.2,97.04 0 top
U17  43.62,86.02 0 top
U18  121.06,86.14 0 top

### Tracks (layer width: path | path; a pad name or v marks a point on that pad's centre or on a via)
+5V  (via drill 0.7)
  Top 0.305: U17.8 44.52,86.02 42.12,83.62 | 11.12,83.62 10.5,84.25 | U15.8 116.88,99.75 116.88,89 116.88,88.62 118.36,87.14 U18.1 120.98,87.14 122,86.12 123.19,86.12 U18.8
  Top 0.61: R1.2 15.28,36.27 15.02,36 | 42.12,83.62 33.25,83.62 | 33.25,83.62 11.12,83.62 | 113.5,143.98 113.09,144.39 R52.2 R51.2 | C18.1 116.86,88.99 116.88,89 | C17.1 33.26,83.64 33.25,83.62
  Top 0.813: 46.5,19.75 v32.62,19.75 32.5,19.62 | 46.5,19.75 v65.62,19.75 77,19.75 | 19.38,19.62 15.02,23.98 15.02,36 LED1.A 10.5,52.27 10.5,84.25 10.5,97 15.02,101.52 LED7.A | LED2.A 46.77,36.12 | 46.77,36.12 46.77,20.02 46.5,19.75 | R6.2 46.91,36.27 46.77,36.12 | LED3.A 77.23,35.88 | 77.23,35.88 77.23,19.98 77,19.75 | R11.2 77.61,36.25 77.23,35.88 | 77,19.75 v98.88,19.75 106.62,19.75 | 106.59,19.71 106.62,19.75 | 106.62,19.75 111,19.75 | 111,19.75 v131.5,19.75 142,19.75 | LED4.A 111.11,36.12 | 111.11,36.12 111.11,19.86 111,19.75 | R16.2 111.23,36.25 111.11,36.12 | 145.75,19.75 v159.38,19.75 169.25,19.75 | 145.75,19.75 142,19.75 | 145.7,19.8 145.75,19.75 | LED5.A 141.85,36.12 | 141.85,36.12 141.85,19.89 142,19.75 | R21.2 141.98,36.25 141.85,36.12 | v189.88,19.75 169.25,19.75 | LED6.A 169.6,36.38 | 169.6,36.38 169.6,20.11 169.25,19.75 | R26.2 169.73,36.25 169.6,36.38 | LED8.A 69.23,101.52 68,102.75 60.5,102.75 | 60.5,102.75 43.55,102.75 U14.8 | 84.83,144 U8.J2.2 84.83,165.15 LCD1.2 | 84.83,144 84.83,136.82 60.75,112.75 60.75,103 60.5,102.75 | U8.J1.1 113.5,143.98 84.84,143.98 84.83,144
  Top 1.27: 19.38,19.62 32.5,19.62 | J1.1 106.59,19.71
  Bottom 0.61: Q1.3 30.25,22.78 R2.2 | J1.1 106.59,10.96 C1.1 | C14.1 41.62,100.82 U14.8 | C15.1 118.5,98.12 U15.8 | U16.8 175.65,100.85 179,97.5 179,95.79 C16.1
  Bottom 0.813: Q1.3 32.55,19.82 v32.62,19.75 | v65.62,19.75 65.56,19.82 Q2.3 63.12,19.97 63.12,21.88 62.02,22.98 R7.2 | v98.88,19.75 98.64,19.52 Q3.3 96.42,22.63 R12.2 | v131.5,19.75 131.26,19.52 Q4.3 129.04,22.63 R17.2 | v159.38,19.75 159.09,19.47 Q5.3 156.72,23.32 R22.2 | v189.88,19.75 189.47,19.34 Q6.3 186.66,23.76 R27.2 | LED8.A 92.38,101.52 | 92.38,101.52 LED9.A 115.11,101.52 U15.8 117.75,103 119.5,104.75 141.38,104.75 144.6,101.52 LED10.A 168.75,101.52 LED11.A 170.35,103.12 170.38,103.12 171.38,104.12 175.25,104.12 | M2.J2.4 92.6,101.75 92.38,101.52 | LED12.A 202.6,101.52 200,104.12 175.25,104.12 | U16.8 175.39,103.98 175.25,104.12 | LED7.A 33.38,101.52 | 33.38,101.52 41.16,101.52 U14.8 | R31.2 33.24,101.66 33.38,101.52
  pour Top: 29.5,100.5 15.5,100.5 12,97 12,53 16,49 16,25 20,21 191.5,21 192,20.5 192,19 191.5,18.5 19,18.5 14,23.5 14,47 9,52 9,96.5 15,102.5 30,102.5 30.5,102 30.5,101 30,100.5
  pour Top (isolate 0.406): 105.5,19 105.5,12 106,11.5 107.5,11.5 108,12 108,19
A1  (via drill 0.7)
  Top 0.305: v36.5,85 41.45,85 U17.5
  Bottom 0.61: G1.+ 23.91,55.84 29.88,49.88 29.88,47.91 U2.3 | G3.+ 29.28,80.78 33.5,85 v36.5,85
  Bottom 0.813: G1.+ G2.+ G3.+ 23.89,80.8 C3.+ 19.52,86.55 Q8.2 Q8.4
A2  (via drill 0.7)
  Top 0.305: U17.6 47.85,85.02 v48.38,84.5
  Bottom 0.61: U4.3 61.67,49.83 55.62,55.88 55.62,60.43 G4.+ | C5.+ 51.38,82.12 49.12,84.38 48.5,84.38 v48.38,84.5
  Bottom 0.813: G4.+ G5.+ G6.+ | C5.+ 55.62,80.75 G6.+ | Q10.4 Q10.2 59.25,84.38 G6.+
A3
  Top 0.305: U17.7 51.73,85.52 51.75,85.5
  Top 0.61: G9.+ 84.69,85.52 84.67,85.5 51.75,85.5
  Bottom 0.61: U6.3 94.19,49.31 | C7.+ 89.38,80.75 G9.+
  Bottom 0.813: 94.19,49.31 94.19,50.06 93.88,50.38 93.88,50.42 89.17,55.12 G7.+ G8.+ 89.17,80.54 G9.+ 89.54,80.79 93.62,84.88 93.62,87.92 Q12.2 Q12.4
A4
  Top 0.305: U18.4 118.02,85.64 117.25,84.88 117.25,81.33 G12.+
  Bottom 0.813: U9.3 126.94,49.31 117.75,58.5 117.75,60.49 G10.+ G11.+ G12.+ | C9.+ 117.75,80.75 G12.+ | G12.+ 120.75,83.75 134.25,83.75 135.12,84.62 Q14.2 Q14.4
A5
  Top 0.305: U18.5 119.98,85.14 122,83.12 144.21,83.12 G15.+
  Bottom 0.305: 140.38,76.38 142.75,78.75 142.75,80.62 C11.+
  Bottom 0.61: Q16.2 Q16.4
  Bottom 0.813: U11.3 155.81,49.19 146.62,58.38 146.62,60.74 G13.+ 146.67,69.54 G14.+ G15.+ | C11.+ 146.5,80.75 G15.+ | G15.+ 146.54,82.05 149.25,84.75 158.62,84.75 159.5,85.62 Q16.2
A6
  Top 0.305: U18.6 125.11,85.14 126.5,83.75 172.21,83.75 G18.+
  Bottom 0.813: 175.29,80.67 G17.+ G16.+ 175.5,60.59 175.5,58 184.44,49.06 U13.3 | 175.29,80.67 G18.+ 175.13,80.75 C13.+ | Q18.4 Q18.2 193.75,86.65 193.75,85.38 192.75,84.38 177.62,84.38 175.29,82.05 175.29,80.67
D1  (via drill 1)
  Top 0.61: M2.J1.1 92.16,135.25 156.5,135.25 201,90.75 205.5,90.75 v205.62,90.62
  Bottom 0.61: Q17.2 202.66,90.54 R49.1 205.58,90.58 v205.62,90.62
D2  (via drill 1)
  Top 0.61: v176.62,97.5 175.75,97.5 172.75,100.5 172.75,116.5 155.25,134 101.07,134 M2.J1.5
  Bottom 0.61: Q15.2 168.85,90.93 R48.1 175.2,90.95 176.62,92.38 v176.62,97.5
D3  (via drill 0.7)
  Top 0.61: v135.38,97.12 135.38,127.12 129.5,133 102.61,133 M2.J1.6
  Bottom 0.61: R47.1 144.8,90.95 143.38,92.38 140.12,92.38 v135.38,97.12
  Bottom 0.813: Q13.2 144.85,90.93 R47.1
D4  (via drill 0.7)
  Top 0.51: 106.62,111.12 106.62,123.62 109.12,126.12 109.12,129 108.12,130 102.15,130 M2.J1.7
  Top 0.61: 106.62,111.12 106.62,109.62 104.5,107.5 v104.5,89.25
  Bottom 0.61: R46.1 102.38,89.25 v104.5,89.25
  Bottom 0.813: Q11.2 102.35,90.8 R46.1
D5  (via drill 1)
  Top 0.61: v74.75,92.12 74.75,106.5 83.38,115.12 91.75,115.12 102.75,126.12 M2.J1.8
  Bottom 0.61: Q9.2 69.1,90.93 R45.1 73.7,91.08 v74.75,92.12
D6  (via drill 1)
  Top 0.51: 99,110.62 99,119.62 105.25,125.88 105.25,128.02 M2.J1.9
  Top 0.61: v89.62,103.88 92.25,103.88 99,110.62
  Bottom 0.61: Q7.2 29.16,90.99 R44.1 41.83,91.08 43,92.25 43,102.38 44.5,103.88 v89.62,103.88
D7
  Bottom 0.813: M2.J1.10 105.36,130.55 SW2.1 SW2.2
D8
  Top 0.61: U1.2 30.25,46.01 40.25,56 40.25,66.25 48.12,74.12 100.88,74.12 105.88,79.12 105.88,106.88 109.12,110.12 109.12,117.38 110.38,118.63 M2.J1.11
D9
  Top 0.406: 111.62,117.5 111.62,110.5 110.12,109
  Top 0.61: U3.2 62.64,45.14 73.5,56 73.5,67.62 78.88,73 101.75,73 107.12,78.38 107.12,106 110.12,109 | 111.62,117.5 112.75,118.62 112.75,127.9 M2.J1.12
D10
  Top 0.406: 114.25,111.88 114.25,117 114.12,117.12
  Top 0.51: 114.25,117.25 114.12,117.12
  Top 0.61: U5.2 95.14,44.52 106.75,56.12 106.75,75.88 108.19,77.31 108.12,77.38 108.12,105.62 114.25,111.75 114.25,111.88 | M2.J1.13 115.46,118.46 114.25,117.25
D11
  Top 0.51: 116.75,117 116.75,112 109.12,104.38 109.12,58 113.38,53.75
  Top 0.61: U7.2 127.77,39.35 113.38,53.75 | M2.J1.14 118,118.25 116.75,117
D12
  Top 0.51: M2.J1.15 119.25,126.78 119.25,111.75 110,102.5 110,59 114.62,54.38
  Top 0.61: U10.2 155.4,45.85 148.88,52.38 116.62,52.38 114.62,54.38 114.38,54.62
D13
  Top 0.61: U12.2 185.4,42.23 173.62,54 117.75,54 115.75,56 115.62,56 111.12,60.5 111.12,102 120.5,111.38 120.5,112.79 M2.J2.15
GND  (via drill 0.7)
  Top 0.305: U17.3 41.45,86 v39.5,86 39.5,87 39.52,87.02 U17.1 | U18.3 117.27,86.14 v116.38,86.12
  Top 0.61: C18.2 116.31,86.19 v116.38,86.12 | C17.2 37.61,87.89 v39.5,86
  Bottom 0.305: v39.5,86 39,86 | v116.38,86.12 116.12,86.12 115.38,85.38
  Bottom 0.61: U2.2 28.98,46.89 29.38,46.5 31.25,46.5 31.5,46.75 31.5,47.25 32,47.75 33.27,47.75 R3.1 | U4.2 60.73,47.02 61.12,46.62 62.75,46.62 64,47.88 65.14,47.88 R8.1 | U6.2 93.25,46.88 93.62,46.5 95.12,46.5 95.5,46.88 95.5,47.88 96.83,47.88 R13.1 | U9.2 126,47.12 126.5,46.62 128.38,46.62 128.62,46.88 128.62,47.88 128.75,48 130.2,48 R18.1 | U11.2 154.88,47.12 155.38,46.62 156.75,46.62 158,47.88 159.33,47.88 R23.1 | U13.2 183.5,46.88 183.88,46.5 185.38,46.5 185.88,47 185.88,47.12 186.75,48 187.95,48 R28.1 | 43.75,76.25 47.25,76.25 48.25,77.25 48.25,80.62 C5.-
  pour Bottom (isolate 0.61): 2,174 224,175 223,0 1,-1
IREG  (via drill 1)
  Top 0.305: U17.4 42.77,85.52 43.5,86.25 43.5,90 U14.3
  Top 0.61: U15.3 120.75,93.33 120.75,95 123.31,97.56 U15.5 | U16.3 180.47,96.09 180.5,96.12 | U16.5 183.12,100.73 183.12,98.12 181.12,96.12 180.5,96.12 | v139.5,96.12 180.5,96.12 | U14.3 46.82,97.12 46.82,98.4 U14.5
  Top 0.813: 46.82,97.12 46.7,97 41.25,97 22.5,115.75 RV1.3
  Bottom 0.61: U14.5 64.31,100.94 65,100.25 111.25,100.25 115.88,95.62 118.46,95.62 U15.3 | U15.5 134.69,100.94 v139.5,96.12
N$1
  Top 0.61: U8.J2.14 115.31,165.15 LCD1.14
N$2
  Top 0.61: U8.J2.13 112.77,165.15 LCD1.13
N$3
  Top 0.61: U8.J2.12 110.22,165.15 LCD1.12
N$4
  Top 0.61: U8.J2.11 107.69,165.15 LCD1.11
N$5
  Top 0.61: U8.J2.6 94.98,165.15 LCD1.6
N$6
  Top 0.61: U8.J2.5 92.44,165.15 LCD1.5
N$7
  Top 0.61: U8.J2.4 89.91,165.15 LCD1.4
N$8
  Bottom 0.813: M2.J1.2 87.5,128.05 87.5,126.5 76.55,115.55 SW1.1 SW1.2
N$9
  Top 0.61: R1.1 27.65,36.27 U1.1
N$10
  Top 0.61: U8.J2.3 87.36,165.15 LCD1.3
N$11
  Bottom 0.61: R30.2 172.27,47.88 LED6.K
N$12
  Bottom 0.61: Q1.1 25.18,22.78 R2.1
  Bottom 0.813: R2.1 26.29,27.29 U1.4
N$13
  Bottom 0.61: Q1.2 27.71,9 | 29.88,45.07 U2.4 33.38,45.12 R3.2 36.53,45.07 C2.+ | 29.12,43.25 29.12,43.12 29,43
  Bottom 1.016: 29,43 20.5,34.5 20.5,10.5 25.25,10.5 25.73,10.98 | 25,11.5 25.21,11.5 25.73,10.98 | 25.73,10.98 27.71,9 | 29.12,43.25 29.25,43.25 29.75,43.75 29.75,44.94 U2.4
N$14
  Bottom 0.61: U2.1 23.52,47.86 R5.1
N$15
  Bottom 0.61: U2.5 23.45,45.12 R4.2
N$16
  Bottom 0.61: R5.2 LED1.K
N$18
  Top 0.813: R6.1 60.03,36.27 U3.1
N$20
  Bottom 0.813: Q2.1 58.07,22.79 R7.1 59.18,27.79 U3.4
N$21
  Bottom 0.61: Q2.2 60.61,10.75 | U4.4 65.18,45.12 R8.2 68.36,45.07 C4.+
  Bottom 1.016: U4.4 61.67,43.92 52.75,35 52.75,10.5 60.36,10.5 60.61,10.75
N$22
  Bottom 0.61: R9.2 59.69,45.22 U4.5
N$24
  Bottom 0.61: R10.1 59.69,47.76 U4.1
N$25
  Bottom 0.61: R10.2 LED2.K
N$26
  Top 0.813: U5.1 88.23,36.31 R11.1
N$28
  Bottom 0.813: Q3.1 91.33,22.63 R12.1 92.45,28.47 U5.4
N$29
  Bottom 0.61: U6.4 94.25,45.07 96.86,45.07 R13.2 100.7,45.2 C6.+
  Bottom 1.016: 94.25,45.07 94.25,43.5 85.5,34.75 85.5,10.5 91.46,10.5 Q3.2
N$30
  Bottom 0.61: R14.2 92.19,45.25 U6.5
N$32
  Bottom 0.61: U6.1 R15.1
N$33
  Bottom 0.813: R15.2 LED3.K
N$34
  Top 0.61: R16.1 125.17,36.25 U7.1
N$36
  Bottom 0.813: Q4.1 123.96,22.63 R17.1 125.08,28.54 U7.4
N$37
  Bottom 0.61: 126.88,45.19 U9.4 130.2,45.25 R18.2 134.08,45.2 C8.+
  Bottom 1.016: 126.88,45.19 126.88,42.38 119,34.5 119,15.59 Q4.2
N$38
  Bottom 0.61: R19.2 U9.5
N$40
  Bottom 0.61: R20.1 U9.1
N$41
  Bottom 0.61: R20.2 LED4.K
N$42
  Top 0.61: R21.1 152.79,36.25 U10.1
N$44
  Bottom 0.813: Q5.1 151.65,23.44 R22.1 152.7,28.54 U10.4
N$45
  Bottom 0.61: U11.4 155.88,45.07 159.37,45.07 R23.2
  Bottom 0.813: R23.2 162.7,45.08 C10.+
  Bottom 1.016: 155.88,45.07 155.88,43.38 147.75,35.25 147.75,10.5 150.5,7.75 153.9,7.75 Q5.2
N$46
  Bottom 0.61: U11.5 151.42,45.13 R24.2
N$48
  Bottom 0.61: R25.1 153.68,48.12 U11.1
N$49
  Bottom 0.61: R25.2 LED5.K
N$50
  Top 0.813: R26.1 182.74,36.25 U12.1
N$52
  Bottom 0.813: Q6.1 181.59,23.76 R27.1 182.7,28.36 U12.4
N$53
  Bottom 0.61: U13.4 184.5,45.07 187.87,45.07 R28.2 191.17,45.2 C12.+
  Bottom 0.813: 184.5,45.07 184.5,42 177.5,35 177.5,10.25 179.75,8 184.04,8 Q6.2
N$54
  Bottom 0.61: U13.5 R29.2
N$56
  Bottom 0.61: U13.1 R30.1
N$58
  Bottom 0.813: D2.C 30.36,110.39 R31.1 30.36,110.46 RV1.2
N$59
  Bottom 0.813: D1.C D2.A
N$60
  Bottom 0.61: R32.2 26.25,93.5 27.25,92.5 40.92,92.5 U14.1
N$61
  Bottom 0.61: Q8.1 22.05,86.77 Q7.1 26.32,91 R32.1
N$62  (via drill 0.7)
  Top 0.61: U14.2 44.28,93.03 40.75,89.5 16.5,89.5 v13.75,86.75
  Bottom 0.61: Q8.3 16.75,86.69 | 16.75,86.69 15.06,86.69 15,86.75 | 16.75,86.69 16.69,86.75 v13.75,86.75 10.55,86.75 R33.1
N$64
  Bottom 0.61: R34.2 66.25,94.38 61,99.62 48.75,99.62 48.12,100.25 48.12,101.75 47.5,102.38 45,102.38 44.25,101.62 44.25,100.97 U14.7
N$65
  Bottom 0.813: Q10.1 66.22,88.05 Q9.1 66.27,91.06 R34.1
N$66
  Bottom 0.813: Q10.3 56.95,90.25 54.9,92.3 R35.1 53.12,92.42 53.12,93.5 46.82,99.81 U14.6
N$68
  Bottom 0.61: R36.2 99.62,92.75 100,92.38 114.75,92.38 U15.1
N$69
  Bottom 0.813: Q12.1 99.47,86.92 Q11.1 99.52,90.84 R36.1
N$70  (via drill 0.7)
  Top 0.61: v103.38,84 91.25,83.88 v88.38,86.75
  Bottom 0.61: v103.38,84 110.5,84 118.23,91.73 U15.2 | R37.1 85.33,86.75 v88.38,86.75 88.55,86.92 Q12.3
N$72
  Bottom 0.61: R38.2 142,99.88 138.38,103.5 120.8,103.5 U15.7
N$73
  Bottom 0.813: Q14.1 141.97,86.92 Q13.1 R38.1
N$74
  Bottom 0.61: R39.1 128.25,93.45 U15.6
  Bottom 0.813: Q14.3 132.82,87.3 130.12,90 128.88,90 128.25,90.62 R39.1
N$76
  Bottom 0.61: R40.2 166.08,93.8 167.5,92.38 174.53,92.38 U16.1
N$77
  Bottom 0.61: R40.1 166.01,90.94 Q15.1 165.96,86.81 Q16.1
N$78  (via drill 0.7)
  Top 0.813: v155.5,88 172.7,88 U16.2
  Bottom 0.813: R41.1 155.45,88.05 v155.5,88 156.69,86.81 Q16.3
N$80
  Bottom 0.61: R42.2 199.88,96.38 195.06,101.19 194.25,102 193.62,102.62 179.75,102.62 179.12,102 179.08,102 U16.7
N$81
  Bottom 0.61: Q18.1 Q17.1 199.83,90.53 R42.1
N$82
  Bottom 0.813: R43.1 186,87.8 | 186,87.8 190.38,87.8 Q18.3 | U16.6 180.47,100.53 186,95 186,87.8
N$84
  Bottom 0.61: R45.2 LED8.K
N$85
  Bottom 0.61: R47.2 LED10.K
N$86
  Bottom 0.61: R48.2 LED11.K
N$87
  Bottom 0.61: R49.2 LED12.K
N$90
  Bottom 0.813: LED9.K 102.25,93.8 R46.2
N$91
  Bottom 0.61: R44.2 LED7.K
SCL  (via drill 1)
  Top 0.305: U17.10 75.61,87.02 | 75.61,87.02 75.62,87 | U18.10 123.52,87.14 125.25,88.88 125.25,114.75 v124.12,115.88 | 75.61,87.02 76.77,87.02 100.25,110.5 100.25,112.8 M2.J2.7
  Top 0.61: R51.1 120.33,149.11 U8.J1.3
  Bottom 0.61: M2.J2.7 103.27,115.88 v124.12,115.88 124.12,145.32 U8.J1.3
SDA  (via drill 1)
  Top 0.305: U18.9 124.39,86.64 125.88,88.12 125.88,113 v127.12,114.25 | U17.9 46.98,86.52 47.25,86.25 77.88,86.25 102.62,111 102.62,112.69 M2.J2.8
  Top 0.61: R52.1 120.14,146.76 U8.J1.2
  Bottom 0.406: 118.5,149.25 118.5,149.62 119.12,150.25 123.75,150.25 125.38,148.62
  Bottom 0.61: v127.12,114.25 126.38,114.25 | 126.38,114.25 123.25,114.25 122.62,114.88 104.81,114.88 M2.J2.8 | U8.J1.2 119.86,146.52 118.5,147.88 118.5,149.25 | 125.38,148.62 126.38,147.62 126.38,114.25

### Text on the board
tPlace: RADIOSCH.EU
bPlace: RADIOSCH.EU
